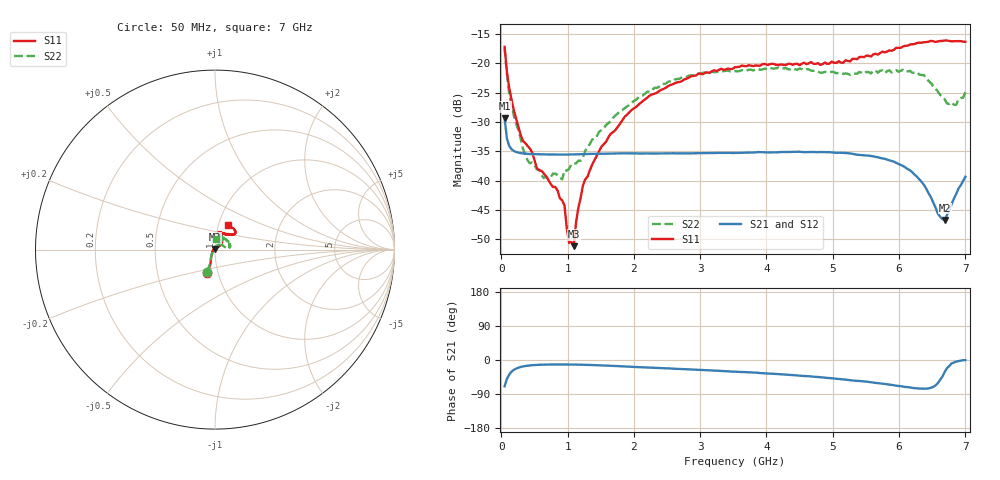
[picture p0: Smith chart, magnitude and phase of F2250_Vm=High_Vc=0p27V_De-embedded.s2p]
! Integrated Device Technology
! Corporate Headquarters
! 6024 Silver Creek Valley Road
! San Jose, CA 95138  USA
! Phone:  1-408-284-8200
! Toll Free:  1-800-223-1366
! Webpage:  http://www.idt.com/
! Timing and RF Division
! 515 Groton Road, Suite 102
! Westford, MA 01886-6024
! Device:  F2250
! Description: Voltage Variable RF Attenuator
! Frequency:  50.0 -  6000.00 MHz
! Package:  3x3 mm Thin QFN Plastic Package: 16 pin
! Ports:  2 RF, 3 DC
!  Pin  1  = GND
!  Pin  2  = NC
!  Pin  3  = RF1  = Port 1
!  Pin  4  = NC
!  Pin  5  = GND
!  Pin  6  = GND
!  Pin  7  = GND
!  Pin  8  = GND
!  Pin  9  = NC
!  Pin 10  = RF2  = Port 2
!  Pin 11  = NC
!  Pin 12  = GND
!  Pin 13  = GND
!  Pin 14  = VCNTRL
!  Pin 15  = VDD
!  Pin 16  = VMODE
! Vcntrl:  0.270 Volts
! Vmode:  +3.300 Volts
! Vdd:  +3.30  Volts
! Current:  1.249 mA
! Data:  The device was measured on a the F2250 evaluation board which has
!  individual transmission lines to the RF pins.  Data was collected
!  using a calibrated network analyzer.  The evaluation board was
!  de-embedded using a TRL calibration technique.
!  The reference plane is the edge of the package pin.
! Misc:  SN 10
!  Action Tracker AT0258
! Date Measured:  2014-11-26
! Date:  2015-10-15  MJV
! Note:
!  Integrated Device Technology supplies this data as a sample of measured
!  data at the package pin for this product.  Your particular data for this
!  product may vary.
!  Data was taken at 25 degrees C.
!  Integrated Device Technology reserves the right to change this data at anytime.
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# GHz S dB R 50
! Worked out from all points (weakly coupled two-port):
!   201 points, 50 MHz to 7 GHz, reference 50 ohm
!   highest |S21| = -29.37 dB at 50 MHz (marker M1); lowest = -46.7 dB at 6.687 GHz (marker M2)
!   lowest |S11| = -51.2 dB at 1.093 GHz (marker M3), VSWR 1.01, Z = 50 + j0.275 ohm
!   |S11| at or under -10 dB: start of sweep to end of sweep
!   |S22| runs from -39.8 to -17.4 dB; largest |S21 - S12| = 5.6e-05
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0.05  -17.18 -108.5  -29.37 -69.4  -29.37 -69.4  -17.41 -110.4
0.08475  -21.47 -107.4  -32.84 -50.0  -32.84 -50.0  -21.93 -108.6
0.15425  -26.23 -116.6  -34.65 -30.9  -34.65 -30.9  -27.21 -119.8
0.29325  -32.27 -127.4  -35.32 -18.4  -35.32 -18.4  -32.90 -132.0
0.3975  -34.12 -142.2  -35.45 -15.0  -35.44 -15.0  -36.57 -157.1
0.5365  -37.88 -154.6  -35.52 -12.9  -35.52 -12.9  -38.08 -179.5
0.64075  -38.77 -162.7  -35.55 -12.2  -35.54 -12.2  -39.58 159.6
0.91875  -43.39 155.9  -35.57 -11.8  -35.57 -11.8  -39.80 124.8
0.9535  -44.25 171.0  -35.57 -11.8  -35.57 -11.8  -38.26 121.5
1.023  -50.63 140.5  -35.56 -11.9  -35.56 -11.9  -38.03 104.7
1.0925  -51.20 88.9  -35.54 -12.0  -35.54 -12.1  -37.06 95.4
1.12725  -47.19 61.4  -35.53 -12.1  -35.53 -12.1  -37.10 88.3
1.2315  -40.85 40.9  -35.49 -12.5  -35.49 -12.5  -36.10 74.0
1.6485  -32.02 41.2  -35.41 -15.2  -35.41 -15.2  -29.91 58.4
2.37825  -24.75 46.7  -35.37 -21.1  -35.37 -21.1  -24.03 53.1
3.525  -20.66 71.7  -35.29 -30.7  -35.30 -30.7  -21.32 72.5
4.7065  -20.06 72.0  -35.13 -44.0  -35.13 -44.0  -21.28 70.1
5.85325  -17.79 40.5  -36.55 -64.9  -36.55 -65.1  -21.18 23.0
6.27025  -16.53 39.4  -39.35 -74.5  -39.36 -74.7  -21.51 8.2
6.68725  -16.11 47.9  -46.75 -31.7  -46.72 -31.5  -26.12 28.1
6.861  -16.22 54.5  -42.30 -4.3  -42.26 -4.2  -27.09 57.5
7  -16.32 62.4  -39.36 -0.4  -39.32 -0.6  -24.90 83.9
